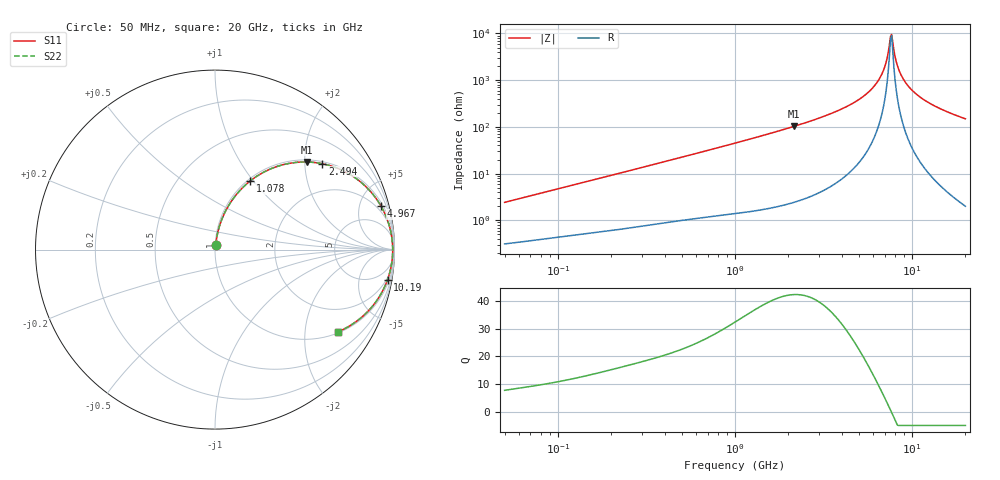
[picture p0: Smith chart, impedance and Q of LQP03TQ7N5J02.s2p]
!Murata Part Number: LQP03TQ7N5J02
!These Parameters are Measured in Series Mode Connection
!  o--[Z]--o
!Port1  Port2
!  o-------o
!Freq. Start=50[MHz] Stop=20[GHz], 401[Steps]
# Hz S RI R 50
!Freq.(Hz) S11(Real) S11(Imag) S21(Real) S21(Imag) S12(Real) S12(Imag) S22(Real) S22(Imag)
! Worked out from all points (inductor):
!   401 points, 50 MHz to 20 GHz, reference 50 ohm
!   read as one part in series: L = 7.59 nH near 51.52 MHz
!   highest Q = 42.3 at 2.147 GHz (marker M1), where L = 7.58 nH
!   self-resonance near 7.554 GHz
!   S11 on the Smith chart (normalised r, x): 50 MHz: 1.01, +0.05; 1.078 GHz: 1.03, +0.97; 2.494 GHz: 1.06, +2.45; 4.967 GHz: 1.33, +7.54; 10.19 GHz: 2, -11; 20 GHz: 1.04, -2.98
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5e7  0.00369 0.0239  0.9963 -0.0239  0.9963 -0.0239  0.00369 0.0239
1.364002e8  0.00892 0.0623  0.9911 -0.0623  0.9911 -0.0623  0.00892 0.0623
3.721004e8  0.0351 0.1605  0.9649 -0.1605  0.9649 -0.1605  0.0351 0.1605
1e9  0.1751 0.3649  0.8249 -0.3649  0.8249 -0.3649  0.1751 0.3649
1.077769e9  0.1972 0.3833  0.8028 -0.3833  0.8028 -0.3833  0.1972 0.3833
2.146657e9  0.5108 0.4882  0.4892 -0.4882  0.4892 -0.4882  0.5108 0.4882
2.493527e9  0.5973 0.4786  0.4027 -0.4786  0.4027 -0.4786  0.5973 0.4786
2.728004e9  0.6492 0.4652  0.3508 -0.4652  0.3508 -0.4652  0.6492 0.4652
3.850025e9  0.8292 0.3615  0.1708 -0.3615  0.1708 -0.3615  0.8292 0.3615
4.966507e9  0.9252 0.2422  0.0748 -0.2422  0.0748 -0.2422  0.9252 0.2422
5.769027e9  0.9622 0.1612  0.0378 -0.1612  0.0378 -0.1612  0.9622 0.1612
6.503449e9  0.9808 0.093  0.0192 -0.093  0.0192 -0.093  0.9808 0.093
7.009217e9  0.9874 0.0495  0.0126 -0.0495  0.0126 -0.0495  0.9874 0.0495
7.442007e9  0.9898 0.0144  0.0102 -0.0144  0.0102 -0.0144  0.9898 0.0144
7.668323e9  0.9901 -0.00319  0.00991 0.00319  0.00991 0.00319  0.9901 -0.00319
7.784049e9  0.99 -0.012  0.01 0.012  0.01 0.012  0.99 -0.012
8.264682e9  0.988 -0.0471  0.012 0.0471  0.012 0.0471  0.988 -0.0471
8.644534e9  0.9849 -0.0734  0.0151 0.0734  0.0151 0.0734  0.9849 -0.0734
9.316812e9  0.9765 -0.1167  0.0235 0.1167  0.0235 0.1167  0.9765 -0.1167
1.019291e10  0.9613 -0.1677  0.0387 0.1677  0.0387 0.1677  0.9613 -0.1677
1.354865e10  0.8771 -0.3159  0.1229 0.3159  0.1229 0.3159  0.8771 -0.3159
2e10  0.6871 -0.457  0.3129 0.457  0.3129 0.457  0.6871 -0.457
